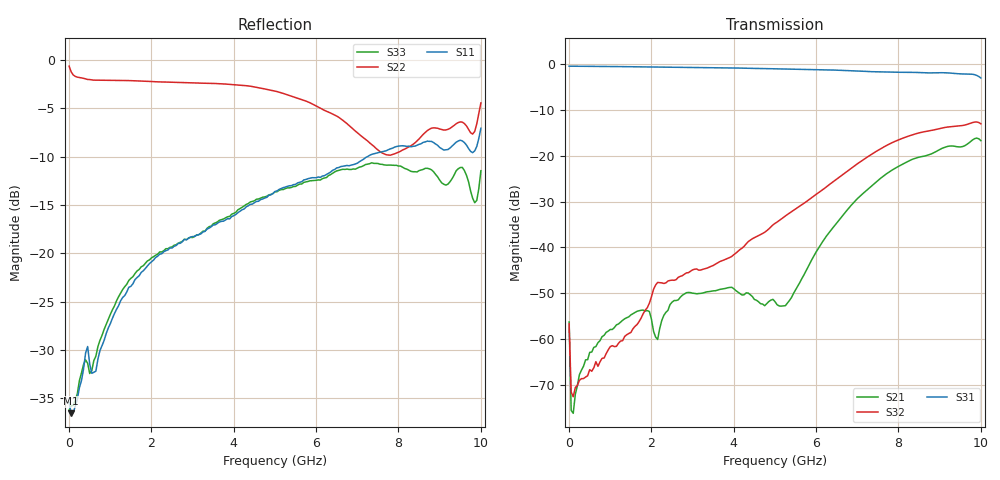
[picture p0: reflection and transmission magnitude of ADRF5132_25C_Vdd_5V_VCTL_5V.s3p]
! Device:  ADRF5132
! Description: Silicon SPDT Switch
! Frequency:  0.7 -  5 GHz
! Ports:
!	RFc	= Port 1
!	RF1	= Port 2
!  RF2  = Port 3
! Vdd:  5 Volt
! Control:  0/5 Volt
! Data:  Data was collected using a calibrated 4 port network analyzer and de-embedded using AtaiTec's In Situ De-Embedding.
! Note:  Analog Devices supplies this data as a sample of measured data
!  for this product.  Your particular data for this product may vary.
!  Data was taken at 25 degrees C.
!  Analog Devices reserves the right to change this data at anytime.
# GHZ S DB R 50.0
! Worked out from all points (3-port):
!   201 points, 10 MHz to 10 GHz, reference 50 ohm
!   strongest paths, dB at 10 MHz, 2.507 GHz, 5.005 GHz, 7.503 GHz, 10 GHz:
!     S31: -0.4, -0.6, -1.0, -1.6, -3.0
!     S32: -56.7, -47.1, -34.7, -18.8, -13.0
!     S21: -56.3, -52.0, -51.8, -25.4, -16.7
!   lowest |S11| = -36.6 dB at 59.95 MHz (marker M1), VSWR 1.03, Z = 51.5 - j0.281 ohm
!   |S11| at or under -10 dB: start of sweep to 7.246 GHz
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0.01  -35.43 -21.8  -57.39 -62.0  -0.41 -0.1
      -56.28 -63.3  -0.64 -8.3  -57.63 -58.2
      -0.40 -0.2  -56.71 -57.6  -36.22 19.1
0.05995  -36.55 -10.6  -74.58 -36.3  -0.41 -1.0
         -75.59 -46.5  -1.23 -42.3  -70.90 -44.0
         -0.41 -1.0  -71.61 -29.1  -35.76 -8.5
0.3097  -33.16 -34.5  -67.00 65.8  -0.40 -4.9
        -66.80 60.6  -1.85 -127.2  -68.96 -38.0
        -0.40 -4.9  -68.66 -38.7  -32.38 -39.1
0.7093  -30.93 -80.6  -60.99 70.3  -0.45 -11.1
        -60.81 71.7  -2.09 -162.1  -65.63 -80.9
        -0.45 -11.1  -65.97 -81.8  -29.64 -68.2
2.15785  -20.30 -137.3  -59.99 81.6  -0.59 -33.2
         -60.10 80.4  -2.26 162.1  -47.63 -139.4
         -0.59 -33.1  -47.64 -139.4  -20.08 -108.7
2.85715  -18.60 -157.5  -49.81 77.7  -0.65 -43.7
         -49.88 77.9  -2.33 151.3  -45.52 -168.1
         -0.66 -43.7  -45.56 -167.9  -18.59 -117.6
5.005  -13.60 162.6  -51.80 2.5  -0.97 -76.7
       -51.83 2.5  -3.22 117.7  -34.74 -176.3
       -0.98 -76.5  -34.74 -176.2  -13.63 -138.7
7.55245  -9.54 117.3  -24.98 160.0  -1.64 -116.4
         -25.00 160.3  -9.48 100.3  -18.51 125.8
         -1.65 -116.1  -18.53 125.8  -10.78 -175.0
9.6004  -8.55 69.9  -17.81 70.3  -2.10 -149.7
        -17.82 70.7  -6.58 97.6  -13.28 49.5
        -2.11 -149.4  -13.28 49.4  -11.44 159.0
10  -7.06 30.5  -16.66 25.7  -2.98 -170.4
    -16.67 26.1  -4.44 25.7  -12.99 22.7
    -2.99 -170.1  -13.00 22.6  -11.45 112.1
